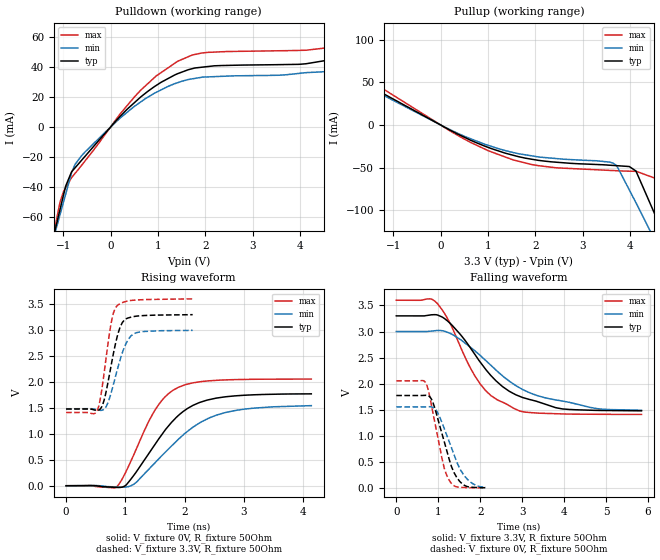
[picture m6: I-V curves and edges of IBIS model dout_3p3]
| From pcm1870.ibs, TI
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|   dout_3p3 Model
[Model]   dout_3p3
Model_type   Output
Polarity   Non-Inverting
Vmeas = 1.65
Vref = 1.65
Cref = 10pF
Rref = 50
|   typ   min   max
C_comp   8.413e-13   6.770e-13   8.859e-13
[Voltage Range]   3.3   3   3.6
|Ambient Temperature   25   85   -40
|Junction Temperature
[Temperature Range]   26   86   -40
[Pullup Reference]   3.3   3   3.6
[Pulldown Reference]   0   0   0
[Power Clamp Reference]   3.3   3   3.6
[GND Clamp Reference]   0   0   0
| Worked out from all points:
|   slope of the pulldown table from 0 to 0.495 V, typ, clamps not added: 30.8 ohm
|   slope of the pullup table from 0 to 0.495 V, typ, clamps not added: 34.7 ohm
|   falling waveform, V_fixture 3.3V, R_fixture 50Ohm: 20-80 % time 1.18ns typ, 1.52ns min, 875ps max; typ from 3.3 V to 1.48 V
|   rising waveform, V_fixture 0V, R_fixture 50Ohm: 20-80 % time 723ps typ, 902ps min, 549ps max; typ from 0 V to 1.77 V
|   rising waveform, V_fixture 3.3V, R_fixture 50Ohm: 20-80 % time 196ps typ, 234ps min, 164ps max; typ from 1.48 V to 3.29 V
|   falling waveform, V_fixture 0V, R_fixture 50Ohm: 20-80 % time 385ps typ, 459ps min, 309ps max; typ from 1.77 V to 0.005 V
[Pulldown]
|   Voltage   I(typ)   I(min)   I(max)
-3.3V     -345.1mA   -312.3mA   -397.2mA
-2.178V   -201.2mA   -186.2mA   -224.6mA
-1.072V   -55.51mA   -58.92mA   -50.67mA
-950.4mV  -39.55mA   -44.97mA   -40.66mA
-822mV    -29.84mA   -30.2mA    -33.69mA
-537mV    -19.43mA   -16.56mA   -22.53mA
638.4mV   20.19mA    16.86mA    24.73mA
1.722V    39.03mA    32.23mA    48.16mA
4.827V    46.01mA    37.51mA    54.64mA
5.524V    49.7mA     42.48mA    61.17mA
6.066V    57.4mA     49.8mA     69.15mA
6.6V      68.92mA    61.29mA    82.02mA
[Pullup]
|   Voltage   I(typ)   I(min)   I(max)
-3.3V     100mA      94.84mA    114.7mA
202.8mV   -6.233mA   -5.556mA   -7.143mA
1.013V    -26.47mA   -24.04mA   -30.36mA
1.528V    -35.42mA   -32.21mA   -40.85mA
2.053V    -41.35mA   -37.32mA   -47.57mA
3.294V    -46.28mA   -41.91mA   -52.46mA
3.642V    -47.38mA   -44.75mA   -53.39mA
3.735V    -47.73mA   -49.5mA    -53.64mA
3.983V    -48.66mA   -76.03mA   -54.12mA
4.122V    -53.87mA   -90.85mA   -54.3mA
4.53V     -105.5mA   -135.9mA   -62.42mA
6.6V      -368.4mA   -364.2mA   -379.8mA
[Ramp]
R_load = 50
|   typ   min   max
dV/dt_r   1.06379/7.2553e-10   0.932857/9.16545e-10   1.23246/5.48889e-10
dV/dt_f   1.09403/1.1878e-09   0.910555/1.53777e-09   1.31417/8.76104e-10
[Falling Waveform]
V_fixture = 3.3V
V_fixture_min = 3V
V_fixture_max = 3.6V
R_fixture = 50Ohm
|   Time   V(typ)   V(min)   V(max)
0s        3.3V       3V         3.6V
934.1ps   3.323V     3.016V     3.572V
1.317ns   3.132V     2.952V     3.102V
1.728ns   2.733V     2.724V     2.362V
2.012ns   2.403V     2.534V     1.982V
2.378ns   2.053V     2.26V      1.706V
2.803ns   1.807V     1.989V     1.526V
3.96ns    1.516V     1.667V     1.42V
4.779ns   1.488V     1.522V     1.413V
5.846ns   1.479V     1.49V      1.411V
[Rising Waveform]
V_fixture = 0V
V_fixture_min = 0V
V_fixture_max = 0V
R_fixture = 50Ohm
|   Time   V(typ)   V(min)   V(max)
0s        476.9pV    23.87nV    444.6pV
853.1ps   -32.43mV   -24.54mV   -26.46mV
1.015ns   15.01mV    -25.09mV   281.2mV
1.191ns   275.6mV    70.72mV    721.8mV
1.497ns   788.5mV    437mV      1.448V
1.666ns   1.063V     635.9mV    1.706V
1.896ns   1.353V     894.1mV    1.895V
2.25ns    1.601V     1.207V     2V
2.699ns   1.713V     1.412V     2.037V
4.139ns   1.769V     1.542V     2.054V
[Rising Waveform]
V_fixture = 3.3V
V_fixture_min = 3V
V_fixture_max = 3.6V
R_fixture = 50Ohm
|   Time   V(typ)   V(min)   V(max)
0s        1.476V     1.482V     1.41V
471.3ps   1.46V      1.477V     1.386V
524.4ps   1.448V     1.464V     1.45V
574ps     1.475V     1.452V     1.651V
643.6ps   1.655V     1.479V     2.183V
773.7ps   2.396V     1.843V     3.207V
873.2ps   2.918V     2.27V      3.477V
985.1ps   3.192V     2.667V     3.539V
1.138ns   3.256V     2.921V     3.571V
2.137ns   3.293V     2.991V     3.597V
[Falling Waveform]
V_fixture = 0V
V_fixture_min = 0V
V_fixture_max = 0V
R_fixture = 50Ohm
|   Time   V(typ)   V(min)   V(max)
0s        1.773V     1.555V     2.054V
711.3ps   1.777V     1.556V     2.004V
838.8ps   1.703V     1.554V     1.588V
973.6ps   1.375V     1.462V     1.037V
1.146ns   882mV      1.135V     373.6mV
1.305ns   439.5mV    796.2mV    96.68mV
1.442ns   199.7mV    500.7mV    21.35mV
1.614ns   56.08mV    241.8mV    9.391mV
1.806ns   13.17mV    90.43mV    4.868mV
2.133ns   4.633mV    11.29mV    2.204mV
